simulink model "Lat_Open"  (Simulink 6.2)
settings: Solver=ode45  StartTime=0.0  StopTime=10.0  RelTol=1e-3
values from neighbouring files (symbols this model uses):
  r2d = 180/pi    (= 57.2957795131)    [run_lat.m]    (also in Pl.m)
undefined symbols (not defined in the file or in its folder): An, Bn, Cn, Dn, Kg

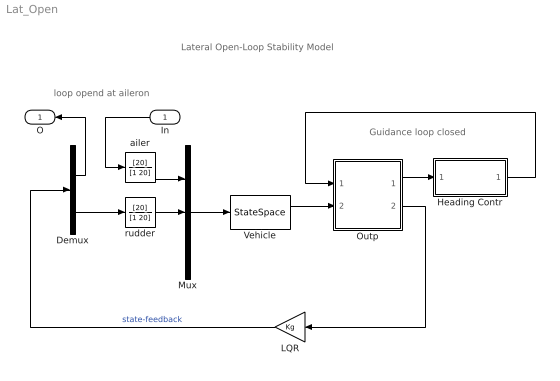
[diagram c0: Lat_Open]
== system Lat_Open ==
  note: Lateral Open-Loop Stability Model
  note: loop opend at aileron
  note: Guidance loop closed
  In : Inport  Orientation=left  Port=1  LatchInput=off
  Demux : Demux  Outputs=2
  Heading Contr : Subsystem
  LQR : Gain  Orientation=left  Gain=Kg  Multiplication=Matrix(K*u) (u vector)
  Mux : Mux  Inputs=3
  Outp : Subsystem
  Vehicle : StateSpace  A=An  B=Bn  C=Cn  D=Dn
  ailer : TransferFcn  Numerator=[20]  Denominator=[1 20]
  rudder : TransferFcn  Numerator=[20]  Denominator=[1 20]
  O : Outport  Orientation=left
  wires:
  Mux/1 -> Vehicle/1
  LQR/1 -> Demux/1  "state-feedback"
  Vehicle/1 -> Outp/2(out)
  ailer/1 -> Mux/1
  rudder/1 -> Mux/2
  Outp/2(x) -> LQR/1
  Outp/1(Vcr) -> Heading Contr/1(Vcr)
  Heading Contr/1(phi-cmd) -> Outp/1(phi-cmd)
  Demux/2 -> rudder/1
  Demux/1 -> O/1
  In/1 -> ailer/1

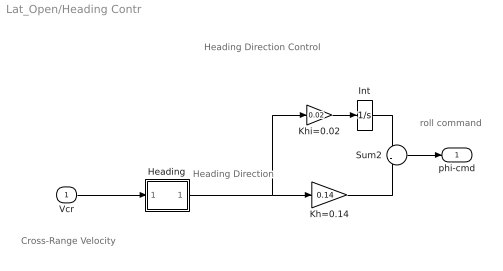
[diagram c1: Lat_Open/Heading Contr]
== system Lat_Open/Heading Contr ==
  note: Cross-Range Velocity
  note: Heading Direction Control
  note: Heading Direction
  note: roll command
  Vcr : Inport  Port=1  LatchInput=off
  Heading : Subsystem
  Int : Integrator
  Kh=0.14 : Gain  Gain=0.14
  Khi=0.02 : Gain  Gain=0.02
  Sum2 : Sum  Inputs=--
  phi-cmd : Outport
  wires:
  Heading/1("chi ") -> Kh=0.14/1, Khi=0.02/1
  Khi=0.02/1 -> Int/1
  Kh=0.14/1 -> Sum2/2
  Int/1 -> Sum2/1
  Sum2/1 -> phi-cmd/1
  Vcr/1 -> Heading/1(Vcr)

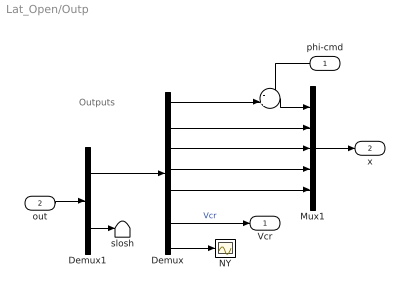
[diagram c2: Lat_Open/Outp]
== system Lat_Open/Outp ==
  note: Outputs
  phi-cmd : Inport  Orientation=left  Port=1  LatchInput=off
  out : Inport  Port=2  LatchInput=off
  "    " : Sum  Inputs=-+|  OutScaling=2^-10
  Demux : Demux  Outputs=7
  Demux1 : Demux  Outputs=[7, 4]
  Mux1 : Mux  Inputs=5
  NY : Scope
  slosh : Terminator
  Vcr : Outport
  x : Outport  Port=2
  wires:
  phi-cmd/1 -> "    "/1
  "    "/1 -> Mux1/1
  Mux1/1 -> x/1
  Demux/6 -> Vcr/1  "Vcr"
  Demux/1 -> "    "/2
  Demux/2 -> Mux1/2
  Demux/3 -> Mux1/3
  Demux/4 -> Mux1/4
  Demux/5 -> Mux1/5
  Demux/7 -> NY/1
  out/1 -> Demux1/1
  Demux1/1 -> Demux/1
  Demux1/2 -> slosh/1

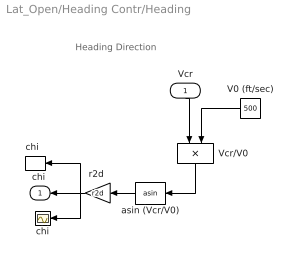
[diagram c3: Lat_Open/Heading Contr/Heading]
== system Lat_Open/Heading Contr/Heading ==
  note: Heading Direction
  Vcr : Inport  Orientation=down  Port=1  LatchInput=off
  V0 (ft/sec) : Constant  Orientation=left  Value=500
  Vcr/V0 : Product  Orientation=down  Inputs=*/
  asin (Vcr/V0) : Trigonometry  Orientation=left  Operator=asin
  chi : Scope
  "chi  " : ToWorkspace  VariableName=chi  SampleTime=-1  SaveFormat=Array
  "r2d " : Gain  Orientation=left  Gain=r2d
  "chi " : Outport  Orientation=left
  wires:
  "r2d "/1 -> "chi "/1, chi/1, "chi  "/1
  Vcr/V0/1 -> asin (Vcr/V0)/1
  asin (Vcr/V0)/1 -> "r2d "/1
  V0 (ft/sec)/1 -> Vcr/V0/2
  Vcr/1 -> Vcr/V0/1
